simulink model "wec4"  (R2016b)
settings: Solver=ode4  StartTime=0  StopTime=1000  FixedStep=0.005  MaxStep=0.005  RelTol=1e-3  EnableMultiTasking=on
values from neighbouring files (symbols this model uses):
  arAdaptiveLawData = 1/2*zModelSimple.zModelPto.arFreq.*     zModelSimple.zModelPto.arMagnitude./     cos(zModelSimple.zModelPto.arPhase*pi/180+pi/2)    [IMPACT_Control.m]
  arAdaptiveLawDataX = 1/2*zModelSimpleX.zModelPto.arFreq.*         zModelSimpleX.zModelPto.arMagnitude./         cos(zModelSimpleX.zModelPto.arPhase*pi/180+pi/2)    [IMPACT_Control.m]
  arControllerRampGain = [0,0,1,1]    [IMPACT_Control.m]
  arControllerRampTime = [0 rStartRampTime rStartRampTime+rRampTimeLength 8000]    [IMPACT_Control.m]
  arEkfInitialisation = zeros(1,11)    [IMPACT_Control.m]
  arEkfInitialisationX = zeros(1,11)    [IMPACT_Control.m]
  arFrequency = zModelSimple.zModelPto.arFreq    [IMPACT_Control.m]
  arFrequencyRange = zModelSimple.zModelPto.arFreq    [IMPACT_Control.m]
  arFrequencyX = zModelSimpleX.zModelPto.arFreq    [IMPACT_Control.m]
  arImpedance = 1./zModelSimple.zModelPto.arMagnitude./zModelSimple.zModelPto.arFreq    [IMPACT_Control.m]
  arImpedanceX = 1./zModelSimpleX.zModelPto.arMagnitude./zModelSimpleX.zModelPto.arFreq    [IMPACT_Control.m]
  CentralPTOPreload = -1.6113e+07    (= -16113000)    [wecSimInputFile.m]
  F1 = [4.243 2.375 -12.243]    [wecSimInputFile.m]
  F2 = [4.243 -2.375 -12.243]    [wecSimInputFile.m]
  F3 = [-4.243 -2.375 -12.243]    [wecSimInputFile.m]
  F4 = [-4.243 2.375 -12.243]    [wecSimInputFile.m]
  FC = [0 0 -14]    [wecSimInputFile.m]
  iAdaptiveDamping = 0    [wec4IMPACT_Project.m]    (also in IMPACT_Control.m = handles.iAdaptiveDamping; wec1_IMPACT_Project.m; wec2_IMPACT_Project.m; wec3_IMPACT_Project.m)
  iControlType = 2    [wec4IMPACT_Project.m]    (also in IMPACT_Control.m = handles.iControlType; wec1_IMPACT_Project.m = 1; wec2_IMPACT_Project.m = 1; wec3_IMPACT_Project.m = 1)
  iPtoPositionConstraint = 1    [wec4IMPACT_Project.m]    (also in IMPACT_Control.m = handles.iPtoPositionConstraint; wec1_IMPACT_Project.m = 0; wec2_IMPACT_Project.m; wec3_IMPACT_Project.m)
  iSensorNoise = 0    [IMPACT_Control.m]
  m = m+1    (= 2)    [checkParamFile.m]
  PTOrotation = atan((T1(2)-F1(2))/(T1(1)-F1(1)))    [wecSimInputFile.m]
  rCogFloater = -8    [wec4_IMPACT_Model.m]    (also in paramInitial.m = get( handles.edit_rCogFloater, 'String' ); wec1_IMPACT_Model.m = -18; wec2_IMPACT_Model.m = -8.5; wec3_IMPACT_Model.m = -0.7)
  rCogSpar = -36.6    [wec4_IMPACT_Model.m]    (also in paramInitial.m = get( handles.edit_rCogSpar, 'String' ); wec3_IMPACT_Model.m = -21.3; wec3_IMPACT_Model2.m = -21.3)
  rDisplacementLimit = 10.000000    (= 10)    [wec4IMPACT_Project.m]    (also in IMPACT_Control.m = getValue(handles.edit_displacementLimit); wec1_IMPACT_Project.m; wec2_IMPACT_Project.m; wec3_IMPACT_Project.m = 3)
  rDisplacementLimitX = 10.000000    (= 10)    [wec4IMPACT_Project.m]    (also in IMPACT_Control.m = getValue(handles.edit_displacementLimitX); wec1_IMPACT_Project.m = 0; wec2_IMPACT_Project.m; wec3_IMPACT_Project.m = 0)
  rGainForAntiWIndUp = tfControllerDiscrete.rGain    [IMPACT_Control.m]
  rGainForAntiWIndUpX = tfControllerXDiscrete.rGain    [IMPACT_Control.m]
  rMaxForcePto = 300000000.000000    (= 300000000)    [wec4IMPACT_Project.m]    (also in IMPACT_Control.m = getValue(handles.edit_maxForcePto); wec1_IMPACT_Project.m = 1e+15; wec2_IMPACT_Project.m = 1e+15; wec3_IMPACT_Project.m = 1000000000)
  rMinForcePto = -300000000.000000    (= -300000000)    [wec4IMPACT_Project.m]    (also in IMPACT_Control.m = getValue(handles.edit_minForcePto); wec1_IMPACT_Project.m = -1e+15; wec2_IMPACT_Project.m = -1e+15; wec3_IMPACT_Project.m = -1000000000)
  rMooringX = 20000    [wec4_IMPACT_Model.m]    (also in paramInitial.m = get( handles.edit_rMooringX, 'String' ); wec3_IMPACT_Model.m = 10000; wec3_IMPACT_Model2.m = 10000)
  rMooringZ = 10000    [wec4_IMPACT_Model.m]    (also in paramInitial.m = get( handles.edit_rMooringZ, 'String' ); wec3_IMPACT_Model.m = 0; wec3_IMPACT_Model2.m = 0)
  rOutputSampleTime = 0.010000    (= 0.01)    [wec4IMPACT_Project.m]    (also in IMPACT_Control.m = getValue(handles.edit_outputSampleTime); wec1_IMPACT_Project.m; wec2_IMPACT_Project.m; wec3_IMPACT_Project.m)
  rPassiveDampingGain = -604830.000000    (= -604830)    [wec4IMPACT_Project.m]    (also in IMPACT_Control.m = getValue(handles.edit_gainPLD); wec1_IMPACT_Project.m = -214018.1537; wec2_IMPACT_Project.m = -1948070; wec3_IMPACT_Project.m = -519390)
  rPassiveDampingGainX = -278660.000000    (= -278660)    [wec4IMPACT_Project.m]    (also in IMPACT_Control.m = getValue(handles.edit_gainPLDX); wec1_IMPACT_Project.m = 0; wec2_IMPACT_Project.m = 0; wec3_IMPACT_Project.m = 0)
  rTetherPretension = 1.6113e+07    (= 16113000)    [wec4_IMPACT_Model.m]    (also in paramInitial.m = get( handles.edit_rTetherPretension, 'String' ); wec3_IMPACT_Model.m = 0; wec3_IMPACT_Model2.m = 0)
  rTetherSpring = 500000    [wec4_IMPACT_Model.m]    (also in paramInitial.m = get( handles.edit_rTetherSpring, 'String' ); wec3_IMPACT_Model.m = 0; wec3_IMPACT_Model2.m = 0)
  rUpperFrequencyLimit = EKFFloater.upperFreq    [IMPACT_Control.m]
  rXf = 4.243    [wec4AdditionalParams.m]
  rXs = 16.075    [wec4AdditionalParams.m]
  rYf = 2.375    [wec4AdditionalParams.m]
  rYs = 16.075    [wec4AdditionalParams.m]
  rZf = 4.243    [wec4AdditionalParams.m]
  rZs = 2.4350    (= 2.435)    [wec4AdditionalParams.m]
  rZTetherF = 6    [wec4AdditionalParams.m]
  rZTetherS = 2.4350    (= 2.435)    [wec4AdditionalParams.m]
  s = tf('s')    [wec4_IMPACT_Model.m]    (also in IMPACT_Control.m; wec1_IMPACT_Model.m; wec2_IMPACT_Model.m; wec3_IMPACT_Model.m)
  SidePTO1Preload = PreloadPTOCorner    (= 0)    [wecSimInputFile.m]
  SidePTO2Preload = PreloadPTOCorner    (= 0)    [wecSimInputFile.m]
  SidePTO3Preload = PreloadPTOCorner    (= 0)    [wecSimInputFile.m]
  SidePTO4Preload = PreloadPTOCorner    (= 0)    [wecSimInputFile.m]
  simu = simulationClass()    [wecSimInputFile.m]
  T1 = [16.075 16.075 -34.165]    [wecSimInputFile.m]
  T2 = [16.075 -16.075 -34.165]    [wecSimInputFile.m]
  T3 = [-16.075 -16.075 -34.165]    [wecSimInputFile.m]
  T4 = [-16.075 16.075 -34.165]    [wecSimInputFile.m]
  TC = [0 0 -34.165]    [wecSimInputFile.m]
  waves = waveClass('irregular')    [wecSimInputFile.m]
  Z = magPhaseToComplex(zModelTf)    [IMPACT_Control.m]
undefined symbols (not defined in the file or in its folder): arControllerDiscreteDen, arControllerDiscreteNum, arControllerDiscreteXDen, arControllerDiscreteXNum, arExcForceFloaterDen, arExcForceFloaterNum, arExcForceFloaterXDen, arExcForceFloaterXNum, arExcForceSparDen, arExcForceSparNum, arExcForceSparXDen, arExcForceSparXNum, arFexcFloaterDen, arFexcFloaterNum, arFexcFloaterXDen, arFexcFloaterXNum, arFexcSparDen, arFexcSparNum, arFexcSparXDen, arFexcSparXNum, Body, body, constraint, CTTime, deg, Elements, geometry, IRKB, kg, lenJ, mooring, N, pto, rAccelerationGainFloater, rAccelerationGainFloaterX, rAccelerationGainSpar, rAccelerationGainSparX, rad, rBuoyancyGainFloater, rBuoyancyGainFloaterX, rBuoyancyGainSpar, rBuoyancyGainSparX, rDampingGainFloater, rDampingGainFloaterX, rDampingGainSpar, rDampingGainSparX, Rigid, rMaxFocePto, wec4_float, wec4_reactor, WECSim_Lib, X, Y
libraries: nesl_utility x380, sm_lib x170, vrlib x91, simulink x12, WECSim_Lib x4
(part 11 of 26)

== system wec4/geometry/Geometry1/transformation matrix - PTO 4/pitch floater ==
  x_f : Inport
  phiF : Inport  Port=2
  z_f : Inport  Port=3
  Product{16..19} (4 alike) : Product
  Sum8 : Sum
  Sum9 : Sum  Inputs=+-
  Trigonometric Function8 : Trigonometry
  Trigonometric Function9 : Trigonometry  Operator=cos
  d_xf_phi : Outport
  d_zf_phi : Outport  Port=2
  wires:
  z_f/1 -> Product19/2, Product17/1
  Sum9/1 -> d_zf_phi/1  "d_zf_phi"
  Product16/1 -> Sum9/2
  Product19/1 -> Sum8/2
  Product18/1 -> Sum8/1
  Trigonometric Function9/1 -> Product17/2, Product18/2
  Product17/1 -> Sum9/1
  phiF/1 -> Trigonometric Function8/1, Trigonometric Function9/1
  Trigonometric Function8/1 -> Product19/1, Product16/1
  Sum8/1 -> d_xf_phi/1  "d_xf_phi"
  x_f/1 -> Product18/1, Product16/2

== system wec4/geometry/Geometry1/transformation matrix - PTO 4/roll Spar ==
  y_s : Inport
  theta : Inport  Port=2
  z_s : Inport  Port=3
  Product{8..11} (4 alike) : Product
  Sum4 : Sum
  Sum5 : Sum  Inputs=+-
  Trigonometric Function4 : Trigonometry
  Trigonometric Function5 : Trigonometry  Operator=cos
  d_ys_theta : Outport
  d_zs_theta : Outport  Port=2
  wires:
  y_s/1 -> Product10/2, Product8/1
  Trigonometric Function5/1 -> Product11/2, Product8/2
  Sum5/1 -> d_zs_theta/1  "d_zs_theta"
  Product11/1 -> Sum5/1
  Trigonometric Function4/1 -> Product9/1, Product10/1
  Sum4/1 -> d_ys_theta/1  "d_ys_theta"
  z_s/1 -> Product11/1, Product9/2
  Product10/1 -> Sum5/2
  Product9/1 -> Sum4/2
  Product8/1 -> Sum4/1
  theta/1 -> Trigonometric Function5/1, Trigonometric Function4/1

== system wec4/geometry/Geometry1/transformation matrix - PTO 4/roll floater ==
  y_f : Inport
  thetaF : Inport  Port=2
  z_f : Inport  Port=3
  Product{12..15} (4 alike) : Product
  Sum6 : Sum  Inputs=+-
  Sum7 : Sum
  Trigonometric Function6 : Trigonometry
  Trigonometric Function7 : Trigonometry  Operator=cos
  d_yf_theta : Outport
  d_zf_theta : Outport  Port=2
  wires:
  Sum7/1 -> d_zf_theta/1  "d_zf_theta"
  thetaF/1 -> Trigonometric Function7/1, Trigonometric Function6/1
  Trigonometric Function7/1 -> Product14/2, Product13/2
  Product14/1 -> Sum6/1
  Product13/1 -> Sum7/1
  Sum6/1 -> d_yf_theta/1  "d_yf_theta"
  Product15/1 -> Sum6/2
  Product12/1 -> Sum7/2
  Trigonometric Function6/1 -> Product12/1, Product15/1
  z_f/1 -> Product13/1, Product15/2
  y_f/1 -> Product12/2, Product14/1

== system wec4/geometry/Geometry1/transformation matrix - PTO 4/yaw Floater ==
  x_f : Inport
  psiF : Inport  Port=2
  y_f : Inport  Port=3
  Product{2..3,6..7} (4 alike) : Product
  Sum1 : Sum
  Sum3 : Sum  Inputs=+-
  Trigonometric Function1 : Trigonometry
  Trigonometric Function3 : Trigonometry  Operator=cos
  d_xf_psi : Outport
  d_yf_psi : Outport  Port=2
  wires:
  x_f/1 -> Product2/1, Product7/2
  Trigonometric Function1/1 -> Product3/1, Product7/1
  y_f/1 -> Product6/1, Product3/2
  Sum1/1 -> d_xf_psi/1  "d_xf_Psi"
  Product7/1 -> Sum3/2
  Trigonometric Function3/1 -> Product2/2, Product6/2
  Product6/1 -> Sum3/1
  Sum3/1 -> d_yf_psi/1  "d_ys_psi"
  psiF/1 -> Trigonometric Function3/1, Trigonometric Function1/1
  Product2/1 -> Sum1/1
  Product3/1 -> Sum1/2

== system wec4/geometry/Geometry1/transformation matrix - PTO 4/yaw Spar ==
  Xs : Inport
  PsiS : Inport  Port=2
  Ys : Inport  Port=3
  Product{,1,4..5} (4 alike) : Product
  Sum : Sum
  Sum2 : Sum  Inputs=+-
  Trigonometric Function : Trigonometry
  Trigonometric Function2 : Trigonometry  Operator=cos
  d_xs_psi : Outport
  d_ys_psi : Outport  Port=2
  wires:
  Ys/1 -> Product4/1, Product1/2
  Product4/1 -> Sum2/1
  Trigonometric Function/1 -> Product5/1, Product1/1
  Product5/1 -> Sum2/2
  Product/1 -> Sum/1
  Sum/1 -> d_xs_psi/1  "d_xs_psi"
  PsiS/1 -> Trigonometric Function2/1, Trigonometric Function/1
  Trigonometric Function2/1 -> Product4/2, Product/2
  Sum2/1 -> d_ys_psi/1  "d_ys_psi"
  Xs/1 -> Product5/2, Product/1
  Product1/1 -> Sum/2

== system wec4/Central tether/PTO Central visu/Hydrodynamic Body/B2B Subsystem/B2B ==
  CrossCoupling : Subsystem
  vel : Outport
  acc : Outport  Port=2
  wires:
  CrossCoupling/2(acc) -> acc/1
  CrossCoupling/1(vel) -> vel/1

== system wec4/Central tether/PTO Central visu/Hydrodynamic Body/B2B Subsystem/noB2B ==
  vel_in : Inport
  acc_in : Inport  Port=2
  vel : Outport
  acc : Outport  Port=2
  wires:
  acc_in/1 -> acc/1
  vel_in/1 -> vel/1  "x"

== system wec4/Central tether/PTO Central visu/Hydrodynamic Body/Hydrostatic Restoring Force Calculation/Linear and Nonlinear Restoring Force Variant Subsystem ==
  note: 1) Add Subsystem or Model blocks as valid variant choices. 2) You cannot connect blocks at this level. At simulation, connectivity is automatically determined, based on the active variant and port name matching.
  In1 : Inport
  In2 : Inport  Port=2
  "Linear Hydrostatic Restoring Force " : Subsystem  VariantControl=sv_linearHydro
  Nonlinear Hydrostatic Restoring Force : Subsystem  VariantControl=sv_nonlinearHydro
  Out1 : Outport

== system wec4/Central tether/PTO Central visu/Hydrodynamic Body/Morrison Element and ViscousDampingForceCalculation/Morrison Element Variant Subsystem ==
  note: 1) Add Subsystem or Model blocks as valid variant choices. 2) You cannot connect blocks at this level. At simulation, connectivity is automatically determined, based on the active variant and port name matching.
  displacement : Inport
  velocity : Inport  Port=2
  acceleration : Inport  Port=3
  time : Inport  Port=4
  Morrison Element Off : Subsystem  VariantControl=sv_MEOff
  Morrison Element On : Subsystem  Variant=on  VariantControl=sv_MEOn
  morison_force : Outport

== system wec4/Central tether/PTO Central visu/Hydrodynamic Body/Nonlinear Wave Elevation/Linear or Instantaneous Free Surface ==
  note: 1) Add Subsystem or Model blocks as valid variant choices. 2) You cannot connect blocks at this level. At simulation, connectivity is automatically determined, based on the active variant and port name matching.
  In1 : Inport
  In2 : Inport  Port=2
  "Instantaneous Water Free Surface  " : Subsystem  VariantControl=sv_instFS
  "Mean Water Free Surface " : Subsystem  VariantControl=sv_meanFS
  Out1 : Outport

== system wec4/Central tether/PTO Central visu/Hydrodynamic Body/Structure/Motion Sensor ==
  note: Measures the position, velocity, and acceleration of the follower (F) frame relative to the base (B) frame. Ouputs a bus of 3 signals, each signal is a vector length 6.
  Angle : MATLAB Function  TreatAsAtomicUnit=on
  Bus Creator : BusCreator  Inputs=3
  Mux : Mux
  Mux1 : Mux  Inputs=6
  Mux2 : Mux  Inputs=6
  PS-Simulink Converter{,1..15} (16 alike) : nesl_utility/PS-Simulink Converter  PhysicalDomain=network_engine_domain  SubClassName=ps_output  LeftPortType=input  RightPortType=output  PseudoPeriodic=off  Frequencies=[]  Unit=1  AffineConversion=off
  Transform Sensor : sm_lib/Frames and Transforms/Transform Sensor  MeasurementFrame=World  SenseAngle=off  SenseAxis=off  SenseAngle1=off  SenseAngle2=off  SenseAngle3=off  SenseQ=on  SenseR=off  SenseOmegaX=on  SenseOmegaY=on  SenseOmegaZ=on  SenseOmega1=off  SenseOmega2=off  SenseOmega3=off  SenseQDot=off  SenseRDot=off  SenseAlphaX=on  SenseAlphaY=on  SenseAlphaZ=on  SenseAlpha1=off  SenseAlpha2=off  SenseAlpha3=off  SenseQDDot=off  SenseRDDot=off  SenseX=on  SenseY=on  SenseZ=on  SenseRad=off  SenseAzim=off  SenseDist=off  SenseInc=off  SenseXDot=on  SenseYDot=on  SenseZDot=on  SenseRadDot=off  SenseAzimDot=off  SenseDistDot=off  SenseIncDot=off  SenseXDDot=on  SenseYDDot=on  SenseZDDot=on  SenseRadDDot=off  SenseAzimDDot=off  SenseDistDDot=off  SenseIncDDot=off
  F : PMIOPort  Port=1  Side=Right
  B : PMIOPort  Port=2  Side=Left
  Response : Outport
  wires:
  PS-Simulink Converter/1 -> Angle/1(Q)
  PS-Simulink Converter4/1 -> Mux2/4  "alphax"
  PS-Simulink Converter10/1 -> Mux1/1  "vx"
  PS-Simulink Converter12/1 -> Mux1/3  "vz"
  PS-Simulink Converter13/1 -> Mux2/1  "ax"
  PS-Simulink Converter14/1 -> Mux2/2  "ay"
  Mux/1 -> Bus Creator/1  "disp"
  Mux1/1 -> Bus Creator/2  "vel"
  Mux2/1 -> Bus Creator/3  "acc"
  Angle/1(E) -> Mux/4
  PS-Simulink Converter7/1 -> Mux/1  "x"
  PS-Simulink Converter8/1 -> Mux/2  "y"
  PS-Simulink Converter9/1 -> Mux/3  "z"
  PS-Simulink Converter5/1 -> Mux2/5  "alphay"
  PS-Simulink Converter6/1 -> Mux2/6  "alphaz"
  PS-Simulink Converter1/1 -> Mux1/4  "omegax"
  PS-Simulink Converter2/1 -> Mux1/5  "omegay"
  PS-Simulink Converter11/1 -> Mux1/2  "vy"
  PS-Simulink Converter3/1 -> Mux1/6  "omegaz"
  PS-Simulink Converter15/1 -> Mux2/3  "az"
  Bus Creator/1 -> Response/1
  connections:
  Transform Sensor/RConn1 -- F/RConn1
  B/RConn1 -- Transform Sensor/LConn1
  Transform Sensor/RConn2 -- PS-Simulink Converter/LConn1
  PS-Simulink Converter15/LConn1 -- Transform Sensor/RConn17
  PS-Simulink Converter14/LConn1 -- Transform Sensor/RConn16
  PS-Simulink Converter13/LConn1 -- Transform Sensor/RConn15
  PS-Simulink Converter12/LConn1 -- Transform Sensor/RConn14
  PS-Simulink Converter11/LConn1 -- Transform Sensor/RConn13
  PS-Simulink Converter10/LConn1 -- Transform Sensor/RConn12
  PS-Simulink Converter9/LConn1 -- Transform Sensor/RConn11
  PS-Simulink Converter8/LConn1 -- Transform Sensor/RConn10
  PS-Simulink Converter7/LConn1 -- Transform Sensor/RConn9
  PS-Simulink Converter4/LConn1 -- Transform Sensor/RConn6
  PS-Simulink Converter5/LConn1 -- Transform Sensor/RConn7
  PS-Simulink Converter6/LConn1 -- Transform Sensor/RConn8
  PS-Simulink Converter1/LConn1 -- Transform Sensor/RConn3
  PS-Simulink Converter2/LConn1 -- Transform Sensor/RConn4
  PS-Simulink Converter3/LConn1 -- Transform Sensor/RConn5

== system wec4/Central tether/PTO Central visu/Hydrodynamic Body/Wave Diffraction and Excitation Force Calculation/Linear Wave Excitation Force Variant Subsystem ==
  note: 1) Add Subsystem or Model blocks as valid variant choices. 2) You cannot connect blocks at this level. At simulation, connectivity is automatically determined, based on the active variant and port name matching.
  In1 : Inport
  Irregular Wave Excitation Force : Subsystem  VariantControl=sv_irregularWaves
  No Wave Excitation Force : Subsystem  VariantControl=sv_noWave
  Regular Wave Excitation Force : Subsystem  VariantControl=sv_regularWaves
  User Defined Wave Excitation Force : Subsystem  VariantControl=sv_udfWaves
  Out1 : Outport

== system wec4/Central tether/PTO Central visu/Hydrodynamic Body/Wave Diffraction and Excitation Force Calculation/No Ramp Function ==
  Action Port : ActionPort
  Constant : Constant
  R : Outport  InitialOutput=1
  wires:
  Constant/1 -> R/1

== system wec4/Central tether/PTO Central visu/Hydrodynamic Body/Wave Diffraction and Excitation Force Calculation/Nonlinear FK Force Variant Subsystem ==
  note: 1) Add Subsystem or Model blocks as valid variant choices. 2) You cannot connect blocks at this level. At simulation, connectivity is automatically determined, based on the active variant and port name matching.
  In1 : Inport
  In2 : Inport  Port=2
  In3 : Inport  Port=3
  No Nonlinear FroudeKrylov Force : Subsystem  VariantControl=sv_linearHydro
  With Nonlinear FroudeKrylov Force : Subsystem  TreatAsAtomicUnit=on  SystemSampleTime=simu.dtNL  VariantControl=sv_nonlinearHydro
  Out1 : Outport

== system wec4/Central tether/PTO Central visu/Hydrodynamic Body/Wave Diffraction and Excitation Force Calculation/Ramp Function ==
  Time : Inport
  Action Port : ActionPort
  Add : Sum
  Add1 : Sum
  Constant : Constant  Value=1/2
  Constant1 : Constant
  Constant2 : Constant  Value=3*pi/2
  Constant3 : Constant  Value=pi
  Divide : Product  Inputs=*/
  Product : Product
  Product1 : Product
  Ramp Time : Constant  Value=simu.rampTime
  Sine Wave Function : Sin  TimeSource=Use external signal  SampleTime=0
  R : Outport
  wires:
  Divide/1 -> Product1/2  "frequency"
  Constant3/1 -> Divide/1
  Product1/1 -> Add1/1
  Add1/1 -> Sine Wave Function/1
  Constant2/1 -> Add1/2  "phase"
  Ramp Time/1 -> Divide/2  "t_ramp"
  Time/1 -> Product1/1  "t"
  Product/1 -> R/1
  Constant/1 -> Product/2
  Constant1/1 -> Add/1
  Sine Wave Function/1 -> Add/2
  Add/1 -> Product/1

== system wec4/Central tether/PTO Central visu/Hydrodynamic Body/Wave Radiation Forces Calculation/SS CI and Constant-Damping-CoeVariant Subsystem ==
  note: 1) Add Subsystem or Model blocks as valid variant choices. 2) You cannot connect blocks at this level. At simulation, connectivity is automatically determined, based on the active variant and port name matching.
  In1 : Inport
  In2 : Inport  Port=2
  Constant Coefficients : Subsystem  VariantControl=sv_constantCoeff
  Convolution Integral Calculation : Subsystem  VariantControl=sv_convolution
  "State-Space Calculation " : Subsystem  VariantControl=sv_stateSpace
  Out1 : Outport

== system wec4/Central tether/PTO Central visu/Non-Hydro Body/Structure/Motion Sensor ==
  note: Measures the position, velocity, and acceleration of the follower (F) frame relative to the base (B) frame. Ouputs a bus of 3 signals, each signal is a vector length 6.
  Angle : MATLAB Function  TreatAsAtomicUnit=on
  Bus Creator : BusCreator  Inputs=3
  Mux : Mux
  Mux1 : Mux  Inputs=6
  Mux2 : Mux  Inputs=6
  PS-Simulink Converter{,1..15} (16 alike) : nesl_utility/PS-Simulink Converter  PhysicalDomain=network_engine_domain  SubClassName=ps_output  LeftPortType=input  RightPortType=output  PseudoPeriodic=off  Frequencies=[]  Unit=1  AffineConversion=off
  Transform Sensor : sm_lib/Frames and Transforms/Transform Sensor  MeasurementFrame=World  SenseAngle=off  SenseAxis=off  SenseAngle1=off  SenseAngle2=off  SenseAngle3=off  SenseQ=on  SenseR=off  SenseOmegaX=on  SenseOmegaY=on  SenseOmegaZ=on  SenseOmega1=off  SenseOmega2=off  SenseOmega3=off  SenseQDot=off  SenseRDot=off  SenseAlphaX=on  SenseAlphaY=on  SenseAlphaZ=on  SenseAlpha1=off  SenseAlpha2=off  SenseAlpha3=off  SenseQDDot=off  SenseRDDot=off  SenseX=on  SenseY=on  SenseZ=on  SenseRad=off  SenseAzim=off  SenseDist=off  SenseInc=off  SenseXDot=on  SenseYDot=on  SenseZDot=on  SenseRadDot=off  SenseAzimDot=off  SenseDistDot=off  SenseIncDot=off  SenseXDDot=on  SenseYDDot=on  SenseZDDot=on  SenseRadDDot=off  SenseAzimDDot=off  SenseDistDDot=off  SenseIncDDot=off
  F : PMIOPort  Port=1  Side=Right
  B : PMIOPort  Port=2  Side=Left
  Response : Outport
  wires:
  PS-Simulink Converter/1 -> Angle/1(Q)
  PS-Simulink Converter4/1 -> Mux2/4  "alphax"
  PS-Simulink Converter10/1 -> Mux1/1  "vx"
  PS-Simulink Converter12/1 -> Mux1/3  "vz"
  PS-Simulink Converter13/1 -> Mux2/1  "ax"
  PS-Simulink Converter14/1 -> Mux2/2  "ay"
  Mux/1 -> Bus Creator/1  "disp"
  Mux1/1 -> Bus Creator/2  "vel"
  Mux2/1 -> Bus Creator/3  "acc"
  Angle/1(E) -> Mux/4
  PS-Simulink Converter7/1 -> Mux/1  "x"
  PS-Simulink Converter8/1 -> Mux/2  "y"
  PS-Simulink Converter9/1 -> Mux/3  "z"
  PS-Simulink Converter5/1 -> Mux2/5  "alphay"
  PS-Simulink Converter6/1 -> Mux2/6  "alphaz"
  PS-Simulink Converter1/1 -> Mux1/4  "omegax"
  PS-Simulink Converter2/1 -> Mux1/5  "omegay"
  PS-Simulink Converter11/1 -> Mux1/2  "vy"
  PS-Simulink Converter3/1 -> Mux1/6  "omegaz"
  PS-Simulink Converter15/1 -> Mux2/3  "az"
  Bus Creator/1 -> Response/1
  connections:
  Transform Sensor/RConn1 -- F/RConn1
  B/RConn1 -- Transform Sensor/LConn1
  Transform Sensor/RConn2 -- PS-Simulink Converter/LConn1
  PS-Simulink Converter15/LConn1 -- Transform Sensor/RConn17
  PS-Simulink Converter14/LConn1 -- Transform Sensor/RConn16
  PS-Simulink Converter13/LConn1 -- Transform Sensor/RConn15
  PS-Simulink Converter12/LConn1 -- Transform Sensor/RConn14
  PS-Simulink Converter11/LConn1 -- Transform Sensor/RConn13
  PS-Simulink Converter10/LConn1 -- Transform Sensor/RConn12
  PS-Simulink Converter9/LConn1 -- Transform Sensor/RConn11
  PS-Simulink Converter8/LConn1 -- Transform Sensor/RConn10
  PS-Simulink Converter7/LConn1 -- Transform Sensor/RConn9
  PS-Simulink Converter4/LConn1 -- Transform Sensor/RConn6
  PS-Simulink Converter5/LConn1 -- Transform Sensor/RConn7
  PS-Simulink Converter6/LConn1 -- Transform Sensor/RConn8
  PS-Simulink Converter1/LConn1 -- Transform Sensor/RConn3
  PS-Simulink Converter2/LConn1 -- Transform Sensor/RConn4
  PS-Simulink Converter3/LConn1 -- Transform Sensor/RConn5

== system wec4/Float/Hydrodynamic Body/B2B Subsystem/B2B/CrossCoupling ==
  note: CrossCoupling block is updated by its mask initialization, which is only called on when a simulation is run. 'From' blocks are automatically created and connected based on the number of bodies in the simulation.
  Mux1 : Mux  Inputs=2
  Mux2 : Mux  Inputs=2
  vel : Outport
  acc : Outport  Port=2
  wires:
  [acc2] -> Mux2/2
  Mux2/1 -> acc/1
  [acc1] -> Mux2/1
  [vel2] -> Mux1/2
  Mux1/1 -> vel/1
  [vel1] -> Mux1/1

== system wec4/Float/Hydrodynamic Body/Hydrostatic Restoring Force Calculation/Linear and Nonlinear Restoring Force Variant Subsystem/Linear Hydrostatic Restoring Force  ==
  In1 : Inport
  Add1 : Sum  Inputs=+-
  Add2 : Sum  Inputs=+++
  Add3 : Sum  Inputs=+-
  Assignment (Add Net Bouyancy Force to Z-Direction) : Assignment  IndexOptions=Index vector (dialog)  Indices=3  OutputSizes=1
  Assignment (Add Net Bouyancy Force to Z-Direction)1 : Assignment  IndexOptions=Index vector (dialog)  Indices=3  OutputSizes=1
  Assignment (Add Net Bouyancy Force to Z-Direction)2 : Assignment  IndexOptions=Index vector (dialog)  Indices=4:6  OutputSizes=1
  Body Mass : Constant  Value=body.hydroForce.storage.mass
  Center of Gravity : Constant  Value=body.cg
  Center of Gravity1 : Constant  Value=body.cb
  Constant1 : Constant  Value=[0 0 0 0 0 0]
  Constant2 : Constant  Value=[0 0 0]
  Cross Product : vrlib/Utilities/Cross Product
  Gravity : Constant  Value=simu.g
  Linear Restioring Coefficient Matrix : Constant  Value=body.hydroForce.linearHydroRestCoef
  Product : Product
  Product1 : Product  Inputs=3
  Product2 : Product  Multiplication=Matrix(*)
  Volume : Constant  Value=body.dispVol
  Water Density : Constant  Value=simu.rho
  Out1 : Outport
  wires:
  Assignment (Add Net Bouyancy Force to Z-Direction)2/1 -> Add2/3
  Constant1/1 -> Assignment (Add Net Bouyancy Force to Z-Direction)/1, Assignment (Add Net Bouyancy Force to Z-Direction)2/1
  Cross Product/1 -> Assignment (Add Net Bouyancy Force to Z-Direction)2/2
  Assignment (Add Net Bouyancy Force to Z-Direction)1/1 -> Cross Product/1
  Constant2/1 -> Assignment (Add Net Bouyancy Force to Z-Direction)1/1
  Add3/1 -> Cross Product/2
  Center of Gravity/1 -> Add3/2  "cg"
  Center of Gravity1/1 -> Add3/1  "x"
  Linear Restioring Coefficient Matrix/1 -> Product2/1  "K"
  Product2/1 -> Add2/2  "Linear Restoring Force"
  Add1/1 -> Assignment (Add Net Bouyancy Force to Z-Direction)/2
  Product1/1 -> Assignment (Add Net Bouyancy Force to Z-Direction)1/2, Add1/2  "F_Buoyancy"
  Product/1 -> Add1/1  "F_Gravity"
  Water Density/1 -> Product1/1  "rho"
  Gravity/1 -> Product/1, Product1/2  "g"
  Volume/1 -> Product1/3  "Vol"
  Add2/1 -> Out1/1  "F_Restoring"
  Assignment (Add Net Bouyancy Force to Z-Direction)/1 -> Add2/1  "Net Buoyancy Force"
  Body Mass/1 -> Product/2  "m"
  In1/1 -> Product2/2  "x"

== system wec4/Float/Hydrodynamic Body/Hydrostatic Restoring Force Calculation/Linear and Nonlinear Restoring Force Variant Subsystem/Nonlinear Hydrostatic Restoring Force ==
  In1 : Inport
  In2 : Inport  Port=2
  Body Mass2 : Constant  Value=body.hydroForce.storage.mass
  Center of Gravity : Constant  Value=body.cg
  Gravity2 : Constant  Value=simu.g
  Rate Transition : RateTransition
  Rate Transition1 : RateTransition
  Restoring Forces : MATLAB Function  TreatAsAtomicUnit=on  SystemSampleTime=simu.dtNL
  STL areas : Constant  Value=body.bodyGeometry.area
  STL centers : Constant  Value=body.bodyGeometry.center
  STL normal vectors : Constant  Value=body.bodyGeometry.norm
  To Workspace1 : ToWorkspace  VariableName=body1_hspressure_out  SaveFormat=Structure With Time  SampleTime=-1
  Water Density1 : Constant  Value=simu.rho
  Out1 : Outport
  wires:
  Rate Transition/1 -> Out1/1
  Restoring Forces/1(f) -> Rate Transition/1
  Rate Transition1/1 -> To Workspace1/1
  Restoring Forces/2(p) -> Rate Transition1/1
  Body Mass2/1 -> Restoring Forces/9(mass)
  STL areas/1 -> Restoring Forces/5(area)
  In2/1 -> Restoring Forces/2(elv)
  STL centers/1 -> Restoring Forces/3(center)
  STL normal vectors/1 -> Restoring Forces/4(tnorm)
  Water Density1/1 -> Restoring Forces/6(rho)
  Gravity2/1 -> Restoring Forces/7(g)  "g"
  Center of Gravity/1 -> Restoring Forces/8(cg)
  In1/1 -> Restoring Forces/1(x)

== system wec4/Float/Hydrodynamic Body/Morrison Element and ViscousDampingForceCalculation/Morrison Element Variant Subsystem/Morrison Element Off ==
  Constant : Constant  Value=[0 0 0 0 0 0]
  morison_force : Outport
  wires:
  Constant/1 -> morison_force/1

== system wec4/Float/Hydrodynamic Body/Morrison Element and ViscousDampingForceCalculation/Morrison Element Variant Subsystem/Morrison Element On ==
  note: 1) Add Subsystem or Model blocks as valid variant choices. 2) You cannot connect blocks at this level. At simulation, connectivity is automatically determined, based on the active variant and port name matching.
  displacement : Inport
  velocity : Inport  Port=2
  acceleration : Inport  Port=3
  time : Inport  Port=4
  Irregular Wave Morison Force : Subsystem  TreatAsAtomicUnit=on  SystemSampleTime=simu.dtME  VariantControl=sv_irregularWaves
  No Wave Morison Force : Subsystem  VariantControl=sv_noWave
  Regular Wave Morison Force : Subsystem  TreatAsAtomicUnit=on  SystemSampleTime=simu.dtME  VariantControl=sv_regularWaves
  morison_force : Outport

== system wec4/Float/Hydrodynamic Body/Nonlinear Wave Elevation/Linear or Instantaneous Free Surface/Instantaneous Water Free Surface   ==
  In1 : Inport
  In2 : Inport  Port=2
  Center of Gravity : Constant  Value=body.cg
  Frequency Spacing : Constant  Value=waves.dw
  Instantaneous FS : MATLAB Function  TreatAsAtomicUnit=on
  Ramp Time : Constant  Value=simu.rampTime
  STL Centers : Constant  Value=body.bodyGeometry.center
  Wave Amplitude : Constant  Value=waves.A
  Wave Direction : Constant  Value=waves.waveDir
  Wave Frequency : Constant  Value=waves.w
  Wave Number : Constant  Value=waves.k
  Wave Random Phase : Constant  Value=waves.phase
  Wave Type Number : Constant  Value=waves.typeNum
  Out1 : Outport
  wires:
  Wave Amplitude/1 -> Instantaneous FS/4(AH)
  Wave Direction/1 -> Instantaneous FS/12(waveDir)
  In1/1 -> Instantaneous FS/1(x)
  In2/1 -> Instantaneous FS/9(t)
  Frequency Spacing/1 -> Instantaneous FS/6(dw)
  Wave Random Phase/1 -> Instantaneous FS/11(phaseRand)
  Ramp Time/1 -> Instantaneous FS/10(rampT)
  Wave Type Number/1 -> Instantaneous FS/8(typeNum)
  Wave Frequency/1 -> Instantaneous FS/5(w)
  Wave Number/1 -> Instantaneous FS/7(k)
  Center of Gravity/1 -> Instantaneous FS/3(cg)
  STL Centers/1 -> Instantaneous FS/2(center)
  Instantaneous FS/1(f) -> Out1/1

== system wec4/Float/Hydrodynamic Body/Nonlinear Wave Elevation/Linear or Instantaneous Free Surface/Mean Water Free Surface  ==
  zero : Constant  Value=0
  Out1 : Outport
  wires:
  zero/1 -> Out1/1

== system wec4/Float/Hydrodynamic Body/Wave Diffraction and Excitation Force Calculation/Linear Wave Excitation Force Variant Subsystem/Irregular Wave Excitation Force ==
  note: Calculates the wave force, F_wave, for the case of Irregular Waves. F_wave = sum( F_wave(i)) where i = each frequency bin.
  In1 : Inport
  Frequency Spacing Delta Omega : Constant  Value=waves.dw  VectorParams1D=off
  Imaginary Part of Wave Excitation : Constant  Value=body.hydroForce.fExt.im  VectorParams1D=off
  MATLAB Function : MATLAB Function  TreatAsAtomicUnit=on
  Random Phase : Constant  Value=waves.phase  VectorParams1D=off
  Real Part of Wave Excitation : Constant  Value=body.hydroForce.fExt.re  VectorParams1D=off
  Wave Frequency : Constant  Value=waves.w  VectorParams1D=off
  Wave Spectrum : Constant  Value=waves.A  VectorParams1D=off
  Out1 : Outport
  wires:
  Frequency Spacing Delta Omega/1 -> MATLAB Function/6(dw)
  In1/1 -> MATLAB Function/7(time)
  Wave Spectrum/1 -> MATLAB Function/1(A)
  Real Part of Wave Excitation/1 -> MATLAB Function/3(fExtRE)
  Imaginary Part of Wave Excitation/1 -> MATLAB Function/4(fExtIM)
  Wave Frequency/1 -> MATLAB Function/2(w)
  MATLAB Function/1(Fext) -> Out1/1
  Random Phase/1 -> MATLAB Function/5(phaseRand)

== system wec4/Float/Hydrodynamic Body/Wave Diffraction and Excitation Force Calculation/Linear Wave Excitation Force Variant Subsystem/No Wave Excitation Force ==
  Constant : Constant  Value=[0 0 0 0 0 0]
  Out1 : Outport
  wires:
  Constant/1 -> Out1/1

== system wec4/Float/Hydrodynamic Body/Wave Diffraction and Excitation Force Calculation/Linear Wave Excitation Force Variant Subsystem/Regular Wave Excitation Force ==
  note: Calculates the wave force, F_wave, for the case of Regular Waves. F_wave = A * cos(w * t) * Re{Fext} - A * sin(w * t) * Im{Fext}
  In1 : Inport
  Add : Sum
  Add1 : Sum  Inputs=+-
  Constant : Constant  Value=pi/2
  Excitation Imaginary Part : Constant  Value=body.hydroForce.fExt.im(1,:)  VectorParams1D=off
  Excitation Real Part : Constant  Value=body.hydroForce.fExt.re(1,:)  VectorParams1D=off
  Product : Product
  Product1 : Product  Inputs=3
  Product2 : Product  Inputs=3
  Sine Wave Function : Sin  TimeSource=Use external signal  SampleTime=0
  Sine Wave Function1 : Sin  TimeSource=Use external signal  SampleTime=0
  Wave Amplitude : Constant  Value=waves.A(1,:)
  Wave Frequency : Constant  Value=waves.w(1,:)
  Out1 : Outport
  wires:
  Constant/1 -> Add/2
  Add/1 -> Sine Wave Function1/1
  Wave Amplitude/1 -> Product1/1, Product2/1  "A"
  Add1/1 -> Out1/1
  Product2/1 -> Add1/2
  Product1/1 -> Add1/1
  Excitation Real Part/1 -> Product1/2  "Re{Fext}"
  Excitation Imaginary Part/1 -> Product2/3  "Im{Fext}"
  Sine Wave Function/1 -> Product2/2  "sin(wt)"
  Sine Wave Function1/1 -> Product1/3  "cos(w*t)"
  Product/1 -> Add/1, Sine Wave Function/1
  Wave Frequency/1 -> Product/2  "w"
  In1/1 -> Product/1  "t"

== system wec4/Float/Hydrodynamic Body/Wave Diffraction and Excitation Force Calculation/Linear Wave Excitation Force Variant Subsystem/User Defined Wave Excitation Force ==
  note: Calculates the wave force, F_wave, for the case of User Defined Waves. F_wave = convolution calculation [1x6]
  InputWaveForceTimeHistory : FromWorkspace  VariableName=[waves.waveAmpTime(:,1),body.hydroForce.userDefinedFe]  SampleTime=0
  Out1 : Outport
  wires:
  InputWaveForceTimeHistory/1 -> Out1/1

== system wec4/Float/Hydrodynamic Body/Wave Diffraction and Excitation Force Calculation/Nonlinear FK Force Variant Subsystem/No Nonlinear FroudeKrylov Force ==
  Constant : Constant  Value=[0 0 0 0 0 0]
  Out1 : Outport
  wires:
  Constant/1 -> Out1/1

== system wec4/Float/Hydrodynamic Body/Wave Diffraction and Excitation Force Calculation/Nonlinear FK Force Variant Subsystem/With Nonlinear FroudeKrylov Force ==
  In1 : Inport
  In2 : Inport  Port=2
  In3 : Inport  Port=3
  Add : Sum  Inputs=+-
  Center of Gravity : Constant  Value=body.hydroData.properties.cg
  Center of Gravity1 : Constant  Value=body.hydroData.properties.cg
  Constant : Constant  Value=[0 0 0]
  Deep Water Flag : Constant  Value=waves.deepWaterWave
  Diffraction and Excitation Forces : MATLAB Function  TreatAsAtomicUnit=on
  Frequency Spacing : Constant  Value=waves.dw
  Gravity : Constant  Value=simu.g
  Mux : Mux  Inputs=2
  STL Areas : Constant  Value=body.bodyGeometry.area
  STL Centers : Constant  Value=body.bodyGeometry.center
  STL Normal Vectors : Constant  Value=body.bodyGeometry.norm
  To Workspace : ToWorkspace  VariableName=body1_wavenonlinearpressure_out  SaveFormat=Structure With Time  SampleTime=-1
  To Workspace1 : ToWorkspace  VariableName=body1_wavelinearpressure_out  SaveFormat=Structure With Time  SampleTime=-1
  Water Density : Constant  Value=simu.rho
  Water Depth : Constant  Value=waves.waterDepth
  Wave Amplitude : Constant  Value=waves.A
  Wave Frequency : Constant  Value=waves.w
  Wave Number : Constant  Value=waves.k
  Wave Random Phase : Constant  Value=waves.phase
  Wave Type Number : Constant  Value=waves.typeNum
  Out1 : Outport
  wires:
  STL Areas/1 -> Diffraction and Excitation Forces/5(area)
  Diffraction and Excitation Forces/2(wp) -> To Workspace/1
  Diffraction and Excitation Forces/3(wpMeanFS) -> To Workspace1/1
  In2/1 -> Add/1
  Constant/1 -> Mux/2
  Center of Gravity/1 -> Mux/1  "cg"
  Mux/1 -> Add/2
  Add/1 -> Diffraction and Excitation Forces/1(x)  "x_cg"
  Deep Water Flag/1 -> Diffraction and Excitation Forces/13(deepWaterWave)
  Wave Random Phase/1 -> Diffraction and Excitation Forces/17(phaseRand)
  Water Depth/1 -> Diffraction and Excitation Forces/12(wDepth)
  Wave Number/1 -> Diffraction and Excitation Forces/14(k)
  Wave Type Number/1 -> Diffraction and Excitation Forces/15(typeNum)
  Frequency Spacing/1 -> Diffraction and Excitation Forces/11(dw)
  Wave Frequency/1 -> Diffraction and Excitation Forces/10(w)
  Wave Amplitude/1 -> Diffraction and Excitation Forces/9(AH)
  In1/1 -> Diffraction and Excitation Forces/16(t)
  In3/1 -> Diffraction and Excitation Forces/2(elv)
  STL Centers/1 -> Diffraction and Excitation Forces/3(center)
  STL Normal Vectors/1 -> Diffraction and Excitation Forces/4(tnorm)
  Water Density/1 -> Diffraction and Excitation Forces/6(rho)
  Gravity/1 -> Diffraction and Excitation Forces/7(g)
  Diffraction and Excitation Forces/1(f) -> Out1/1
  Center of Gravity1/1 -> Diffraction and Excitation Forces/8(cg)

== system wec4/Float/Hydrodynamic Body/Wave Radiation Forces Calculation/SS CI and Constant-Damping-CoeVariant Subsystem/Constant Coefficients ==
  In1 : Inport
  Product : Product  Multiplication=Matrix(*)
  Radiation Damping Matrix : Constant  Value=body.hydroForce.fDamping
  Out1 : Outport
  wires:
  In1/1 -> Product/2
  Product/1 -> Out1/1  "F_Single Frequency"
  Radiation Damping Matrix/1 -> Product/1

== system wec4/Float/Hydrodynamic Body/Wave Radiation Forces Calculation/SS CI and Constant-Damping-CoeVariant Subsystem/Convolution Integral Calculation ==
  In1 : Inport
  MATLAB Function : MATLAB Function  TreatAsAtomicUnit=on  SystemSampleTime=simu.CTTime(2) - simu.CTTime(1)
  Rate Transition : RateTransition
  Reshape : Reshape
  Out1 : Outport
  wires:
  Rate Transition/1 -> Reshape/1
  MATLAB Function/1(F_FM) -> Rate Transition/1
  Reshape/1 -> Out1/1
  In1/1 -> MATLAB Function/1(v)

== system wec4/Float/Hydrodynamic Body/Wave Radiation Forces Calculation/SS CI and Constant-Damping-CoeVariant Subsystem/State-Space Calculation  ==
  In1 : Inport
  State-Space : StateSpace  A=body.hydroForce.ssRadf.A  B=body.hydroForce.ssRadf.B  C=body.hydroForce.ssRadf.C  D=body.hydroForce.ssRadf.D  X0=0
  Out1 : Outport
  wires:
  State-Space/1 -> Out1/1
  In1/1 -> State-Space/1  "x"

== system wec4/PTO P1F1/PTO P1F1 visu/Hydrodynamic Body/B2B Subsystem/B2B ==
  CrossCoupling : Subsystem
  vel : Outport
  acc : Outport  Port=2
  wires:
  CrossCoupling/2(acc) -> acc/1
  CrossCoupling/1(vel) -> vel/1

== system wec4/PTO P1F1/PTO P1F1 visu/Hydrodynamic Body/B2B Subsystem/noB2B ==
  vel_in : Inport
  acc_in : Inport  Port=2
  vel : Outport
  acc : Outport  Port=2
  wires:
  acc_in/1 -> acc/1
  vel_in/1 -> vel/1  "x"

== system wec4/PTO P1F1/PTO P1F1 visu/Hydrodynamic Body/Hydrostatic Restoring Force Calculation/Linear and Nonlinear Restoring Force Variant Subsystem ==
  note: 1) Add Subsystem or Model blocks as valid variant choices. 2) You cannot connect blocks at this level. At simulation, connectivity is automatically determined, based on the active variant and port name matching.
  In1 : Inport
  In2 : Inport  Port=2
  "Linear Hydrostatic Restoring Force " : Subsystem  VariantControl=sv_linearHydro
  Nonlinear Hydrostatic Restoring Force : Subsystem  VariantControl=sv_nonlinearHydro
  Out1 : Outport

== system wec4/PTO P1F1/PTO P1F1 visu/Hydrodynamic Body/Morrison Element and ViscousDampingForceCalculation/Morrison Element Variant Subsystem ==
  note: 1) Add Subsystem or Model blocks as valid variant choices. 2) You cannot connect blocks at this level. At simulation, connectivity is automatically determined, based on the active variant and port name matching.
  displacement : Inport
  velocity : Inport  Port=2
  acceleration : Inport  Port=3
  time : Inport  Port=4
  Morrison Element Off : Subsystem  VariantControl=sv_MEOff
  Morrison Element On : Subsystem  Variant=on  VariantControl=sv_MEOn
  morison_force : Outport

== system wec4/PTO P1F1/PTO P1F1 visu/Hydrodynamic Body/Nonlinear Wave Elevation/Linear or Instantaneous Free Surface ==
  note: 1) Add Subsystem or Model blocks as valid variant choices. 2) You cannot connect blocks at this level. At simulation, connectivity is automatically determined, based on the active variant and port name matching.
  In1 : Inport
  In2 : Inport  Port=2
  "Instantaneous Water Free Surface  " : Subsystem  VariantControl=sv_instFS
  "Mean Water Free Surface " : Subsystem  VariantControl=sv_meanFS
  Out1 : Outport

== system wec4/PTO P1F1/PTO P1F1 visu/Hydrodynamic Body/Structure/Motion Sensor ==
  note: Measures the position, velocity, and acceleration of the follower (F) frame relative to the base (B) frame. Ouputs a bus of 3 signals, each signal is a vector length 6.
  Angle : MATLAB Function  TreatAsAtomicUnit=on
  Bus Creator : BusCreator  Inputs=3
  Mux : Mux
  Mux1 : Mux  Inputs=6
  Mux2 : Mux  Inputs=6
  PS-Simulink Converter{,1..15} (16 alike) : nesl_utility/PS-Simulink Converter  PhysicalDomain=network_engine_domain  SubClassName=ps_output  LeftPortType=input  RightPortType=output  PseudoPeriodic=off  Frequencies=[]  Unit=1  AffineConversion=off
  Transform Sensor : sm_lib/Frames and Transforms/Transform Sensor  MeasurementFrame=World  SenseAngle=off  SenseAxis=off  SenseAngle1=off  SenseAngle2=off  SenseAngle3=off  SenseQ=on  SenseR=off  SenseOmegaX=on  SenseOmegaY=on  SenseOmegaZ=on  SenseOmega1=off  SenseOmega2=off  SenseOmega3=off  SenseQDot=off  SenseRDot=off  SenseAlphaX=on  SenseAlphaY=on  SenseAlphaZ=on  SenseAlpha1=off  SenseAlpha2=off  SenseAlpha3=off  SenseQDDot=off  SenseRDDot=off  SenseX=on  SenseY=on  SenseZ=on  SenseRad=off  SenseAzim=off  SenseDist=off  SenseInc=off  SenseXDot=on  SenseYDot=on  SenseZDot=on  SenseRadDot=off  SenseAzimDot=off  SenseDistDot=off  SenseIncDot=off  SenseXDDot=on  SenseYDDot=on  SenseZDDot=on  SenseRadDDot=off  SenseAzimDDot=off  SenseDistDDot=off  SenseIncDDot=off
  F : PMIOPort  Port=1  Side=Right
  B : PMIOPort  Port=2  Side=Left
  Response : Outport
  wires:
  PS-Simulink Converter/1 -> Angle/1(Q)
  PS-Simulink Converter4/1 -> Mux2/4  "alphax"
  PS-Simulink Converter10/1 -> Mux1/1  "vx"
  PS-Simulink Converter12/1 -> Mux1/3  "vz"
  PS-Simulink Converter13/1 -> Mux2/1  "ax"
  PS-Simulink Converter14/1 -> Mux2/2  "ay"
  Mux/1 -> Bus Creator/1  "disp"
  Mux1/1 -> Bus Creator/2  "vel"
  Mux2/1 -> Bus Creator/3  "acc"
  Angle/1(E) -> Mux/4
  PS-Simulink Converter7/1 -> Mux/1  "x"
  PS-Simulink Converter8/1 -> Mux/2  "y"
  PS-Simulink Converter9/1 -> Mux/3  "z"
  PS-Simulink Converter5/1 -> Mux2/5  "alphay"
  PS-Simulink Converter6/1 -> Mux2/6  "alphaz"
  PS-Simulink Converter1/1 -> Mux1/4  "omegax"
  PS-Simulink Converter2/1 -> Mux1/5  "omegay"
  PS-Simulink Converter11/1 -> Mux1/2  "vy"
  PS-Simulink Converter3/1 -> Mux1/6  "omegaz"
  PS-Simulink Converter15/1 -> Mux2/3  "az"
  Bus Creator/1 -> Response/1
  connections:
  Transform Sensor/RConn1 -- F/RConn1
  B/RConn1 -- Transform Sensor/LConn1
  Transform Sensor/RConn2 -- PS-Simulink Converter/LConn1
  PS-Simulink Converter15/LConn1 -- Transform Sensor/RConn17
  PS-Simulink Converter14/LConn1 -- Transform Sensor/RConn16
  PS-Simulink Converter13/LConn1 -- Transform Sensor/RConn15
  PS-Simulink Converter12/LConn1 -- Transform Sensor/RConn14
  PS-Simulink Converter11/LConn1 -- Transform Sensor/RConn13
  PS-Simulink Converter10/LConn1 -- Transform Sensor/RConn12
  PS-Simulink Converter9/LConn1 -- Transform Sensor/RConn11
  PS-Simulink Converter8/LConn1 -- Transform Sensor/RConn10
  PS-Simulink Converter7/LConn1 -- Transform Sensor/RConn9
  PS-Simulink Converter4/LConn1 -- Transform Sensor/RConn6
  PS-Simulink Converter5/LConn1 -- Transform Sensor/RConn7
  PS-Simulink Converter6/LConn1 -- Transform Sensor/RConn8
  PS-Simulink Converter1/LConn1 -- Transform Sensor/RConn3
  PS-Simulink Converter2/LConn1 -- Transform Sensor/RConn4
  PS-Simulink Converter3/LConn1 -- Transform Sensor/RConn5

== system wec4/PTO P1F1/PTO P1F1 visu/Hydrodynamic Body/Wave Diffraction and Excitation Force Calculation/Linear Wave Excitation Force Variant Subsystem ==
  note: 1) Add Subsystem or Model blocks as valid variant choices. 2) You cannot connect blocks at this level. At simulation, connectivity is automatically determined, based on the active variant and port name matching.
  In1 : Inport
  Irregular Wave Excitation Force : Subsystem  VariantControl=sv_irregularWaves
  No Wave Excitation Force : Subsystem  VariantControl=sv_noWave
  Regular Wave Excitation Force : Subsystem  VariantControl=sv_regularWaves
  User Defined Wave Excitation Force : Subsystem  VariantControl=sv_udfWaves
  Out1 : Outport

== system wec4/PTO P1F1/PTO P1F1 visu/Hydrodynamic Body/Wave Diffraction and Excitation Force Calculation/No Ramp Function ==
  Action Port : ActionPort
  Constant : Constant
  R : Outport  InitialOutput=1
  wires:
  Constant/1 -> R/1

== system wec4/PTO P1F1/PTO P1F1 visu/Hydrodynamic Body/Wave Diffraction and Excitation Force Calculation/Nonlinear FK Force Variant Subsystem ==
  note: 1) Add Subsystem or Model blocks as valid variant choices. 2) You cannot connect blocks at this level. At simulation, connectivity is automatically determined, based on the active variant and port name matching.
  In1 : Inport
  In2 : Inport  Port=2
  In3 : Inport  Port=3
  No Nonlinear FroudeKrylov Force : Subsystem  VariantControl=sv_linearHydro
  With Nonlinear FroudeKrylov Force : Subsystem  TreatAsAtomicUnit=on  SystemSampleTime=simu.dtNL  VariantControl=sv_nonlinearHydro
  Out1 : Outport

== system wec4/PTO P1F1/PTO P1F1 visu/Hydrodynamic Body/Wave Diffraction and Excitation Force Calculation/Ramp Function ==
  Time : Inport
  Action Port : ActionPort
  Add : Sum
  Add1 : Sum
  Constant : Constant  Value=1/2
  Constant1 : Constant
  Constant2 : Constant  Value=3*pi/2
  Constant3 : Constant  Value=pi
  Divide : Product  Inputs=*/
  Product : Product
  Product1 : Product
  Ramp Time : Constant  Value=simu.rampTime
  Sine Wave Function : Sin  TimeSource=Use external signal  SampleTime=0
  R : Outport
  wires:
  Divide/1 -> Product1/2  "frequency"
  Constant3/1 -> Divide/1
  Product1/1 -> Add1/1
  Add1/1 -> Sine Wave Function/1
  Constant2/1 -> Add1/2  "phase"
  Ramp Time/1 -> Divide/2  "t_ramp"
  Time/1 -> Product1/1  "t"
  Product/1 -> R/1
  Constant/1 -> Product/2
  Constant1/1 -> Add/1
  Sine Wave Function/1 -> Add/2
  Add/1 -> Product/1

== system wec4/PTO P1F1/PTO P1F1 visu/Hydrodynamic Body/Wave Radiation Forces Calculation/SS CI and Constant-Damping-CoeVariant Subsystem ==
  note: 1) Add Subsystem or Model blocks as valid variant choices. 2) You cannot connect blocks at this level. At simulation, connectivity is automatically determined, based on the active variant and port name matching.
  In1 : Inport
  In2 : Inport  Port=2
  Constant Coefficients : Subsystem  VariantControl=sv_constantCoeff
  Convolution Integral Calculation : Subsystem  VariantControl=sv_convolution
  "State-Space Calculation " : Subsystem  VariantControl=sv_stateSpace
  Out1 : Outport
